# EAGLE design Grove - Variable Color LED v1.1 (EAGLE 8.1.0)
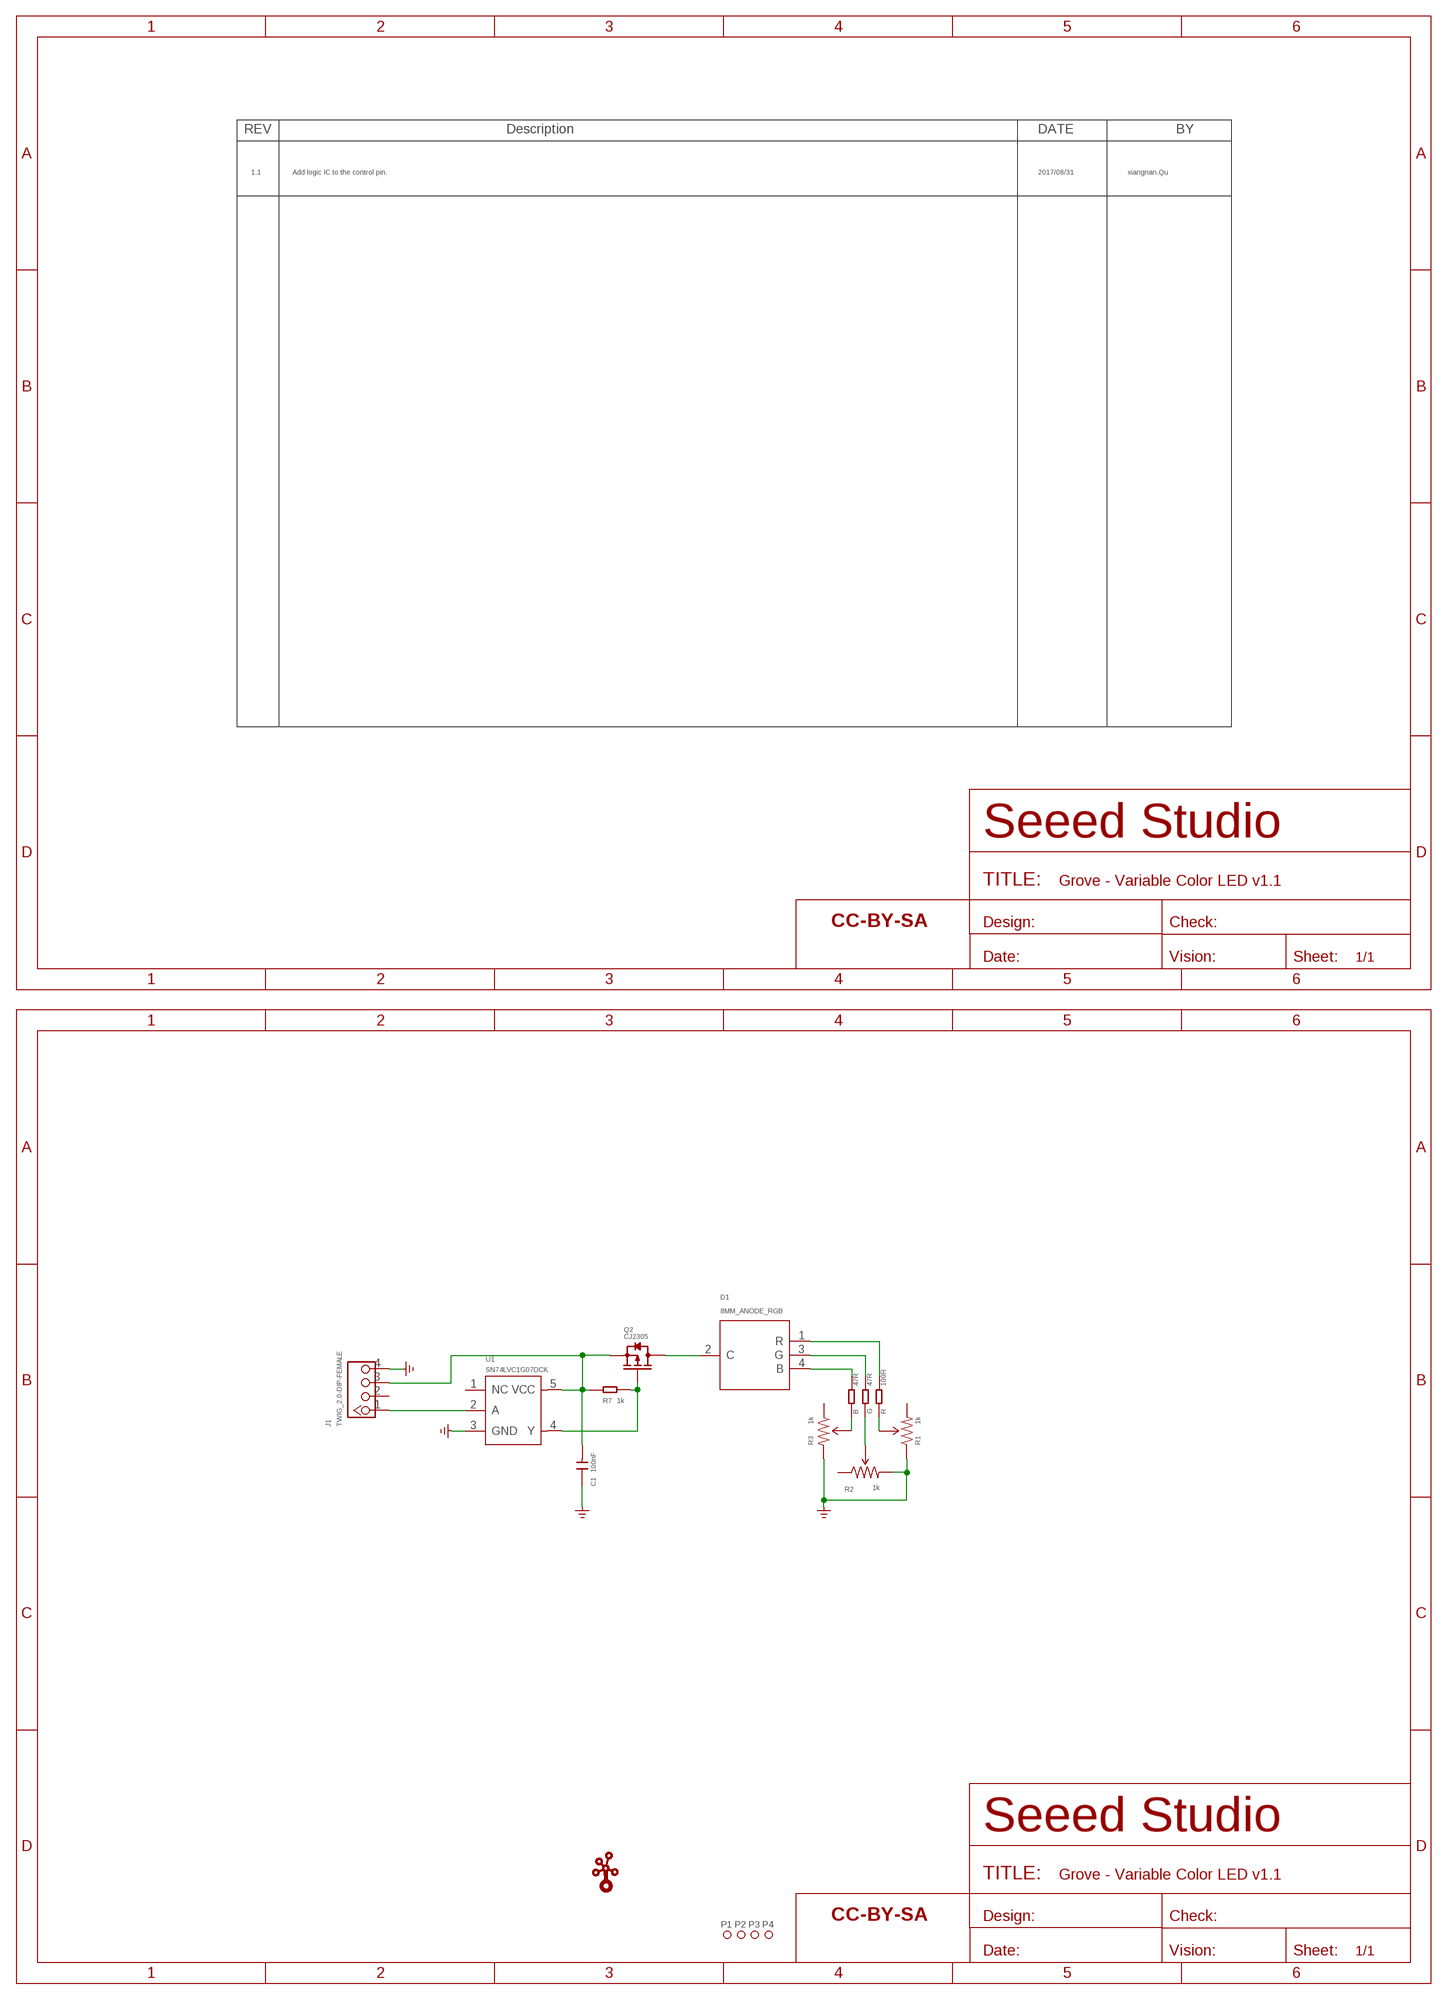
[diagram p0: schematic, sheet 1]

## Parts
B  47R  RES-0402  [R0402]
C1  100nF  CAP-0402  [C0402]
D1  8MM_ANODE_RGB  007-RGB-3P-DIP  [007-RGB-3P-DIP]
FR1  SEEEDSTUDIO-OPEN-SCH-FRAME  [SEEEDSTUDIO-PCB-FRAME]
FR2  SEEEDSTUDIO-OPEN-SCH-FRAME  [SEEEDSTUDIO-PCB-FRAME]
G  47R  RES-0402  [R0402]
J1  TWIG_2.0-DIP-FEMALE  [2.0_1X4]
P1  PAD-MARK'ANNULAR'  [ROUND-MARK-1.0]
P2  PAD-MARK'ANNULAR'  [ROUND-MARK-1.0]
P3  PAD-MARK'ANNULAR'  [ROUND-MARK-1.0]
P4  PAD-MARK'ANNULAR'  [ROUND-MARK-1.0]
Q2  CJ2305  014-P-MOSFETSOT23  [SOT23_]
R  100R  RES-0402  [R0402]
R1  1k  005-TRIMPOTSMD  [TRIMPOT-3MM]
R2  1k  005-TRIMPOTSMD  [TRIMPOT-3MM]
R3  1k  005-TRIMPOTSMD  [TRIMPOT-3MM]
R7  1k  RES-0402  [R0402]
U1  SN74LVC1G07DCK  LOGIC-SN74LVC1G07-DCK  [5P-SMD-2X1.2X1MM]
U$1  TWIGLOGOTWIGLOGO_SMALL  [TWIGLOGO_SMALL]

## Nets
GND: C1.1 J1.4 R1.1(CCW) R2.3(CW) R3.3(CW) U1.3(GND) ; supply symbol labelled GND_POWER
N$1: D1.1(R) R.2
N$2: D1.3(G) G.2
N$3: B.2 D1.4(B)
N$4: G.1 R2.2(WIPER)
N$5: R1.2(WIPER) R.1
N$6: B.1 R3.2(WIPER)
ON/OFF: J1.1 U1.2(A)
RGD_POWER: D1.2(C) Q2.3(D)
SS: Q2.1(G) R7.1 U1.4(Y)
VCC: C1.2 J1.3 Q2.2(S) R7.2 U1.5(VCC)
Unconnected: J1.2 R1.3(CW) R2.1(CCW) R3.1(CCW) U1.1(NC)

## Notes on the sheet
- 1.1 | Add logic IC to the control pin. | 2017/08/31 | xiangnan.Qu

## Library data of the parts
B G R R7 = Discrete-new:RES
C1 = Discrete-new:CAP: Ceramic Capacitors
D1 = Discrete:007-RGB-3P-DIP
FR1 FR2 = moudle-new:SEEEDSTUDIO-OPEN-SCH-FRAME
J1 = Connector:TWIG_2.0-DIP-FEMALE
P1-P4 = Discrete-new:PAD-MARK; PARTNO: DNP
Q2 = Discrete:014-P-MOSFET*: Si2305DS Si2323CDS
R1-R3 = Discrete:005-TRIMPOT
U1 = IC-new:LOGIC-SN74LVC1G07: DRL:310050096 DCK:310050079
U$1 = seeedleo:TWIGLOGO

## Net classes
0 default: width 0.152 mm, drill 0.203 mm, clearance 0.152 mm

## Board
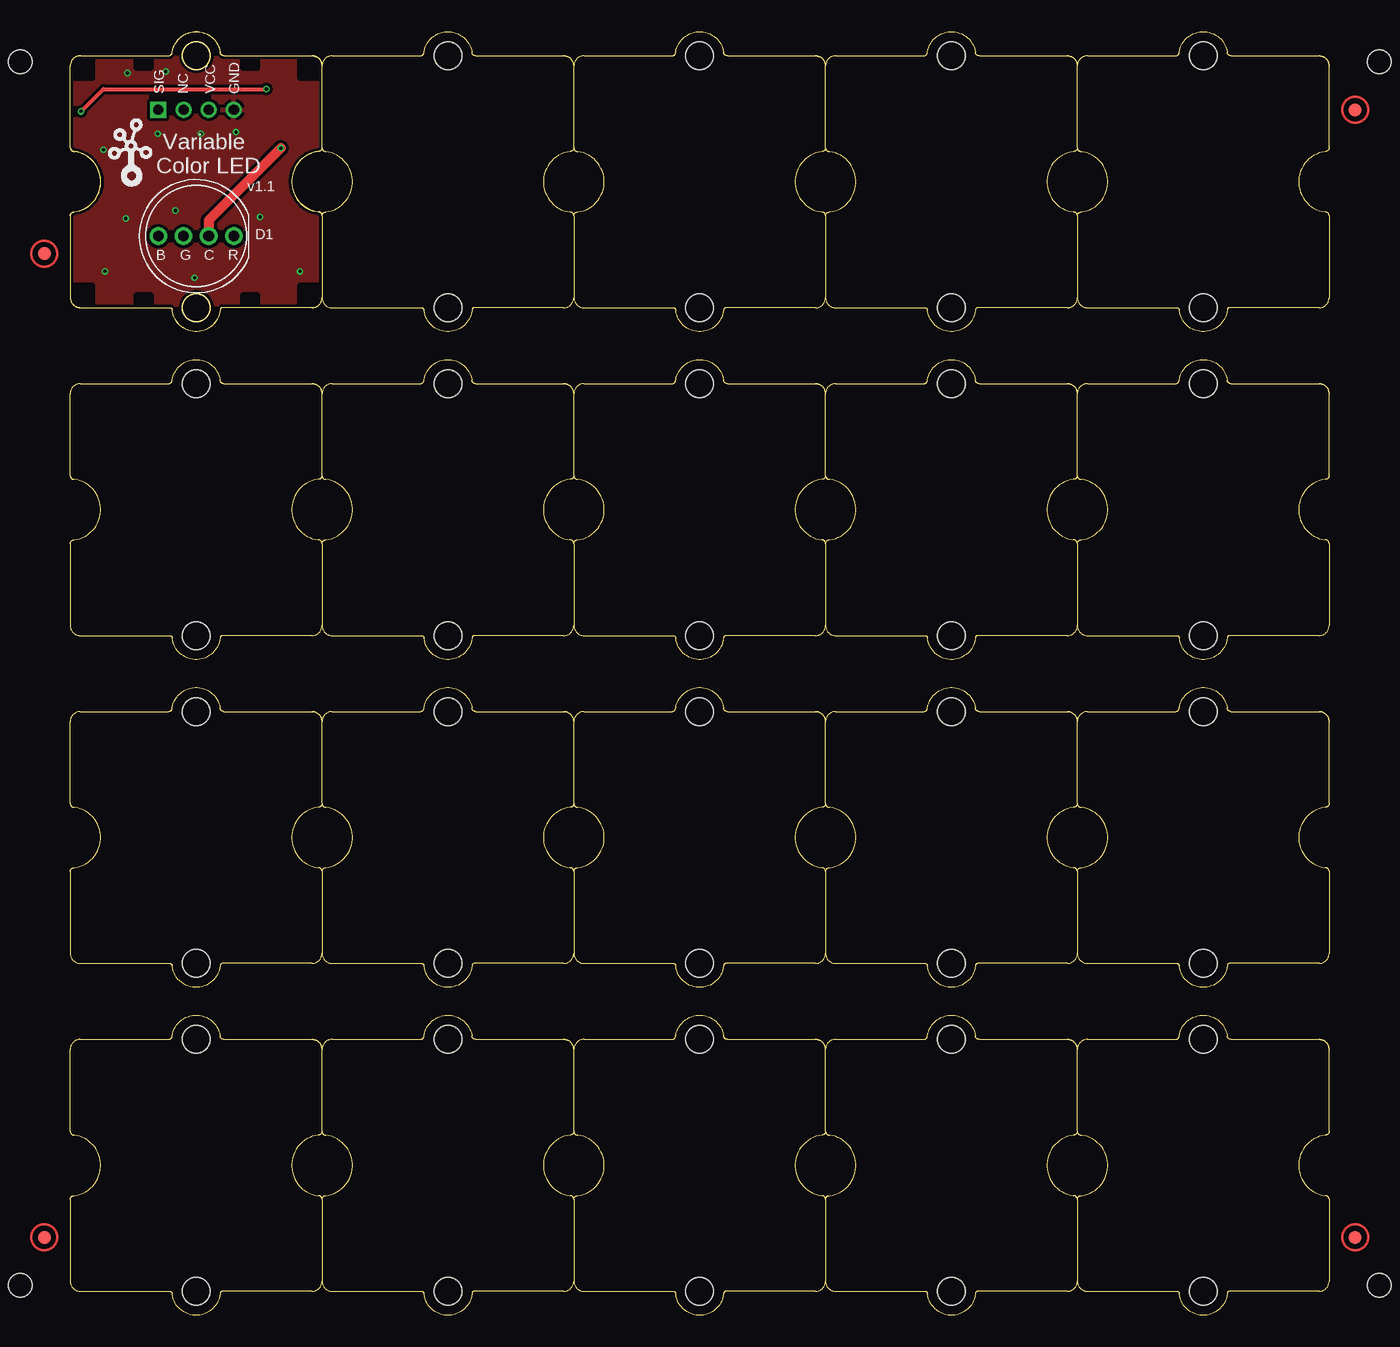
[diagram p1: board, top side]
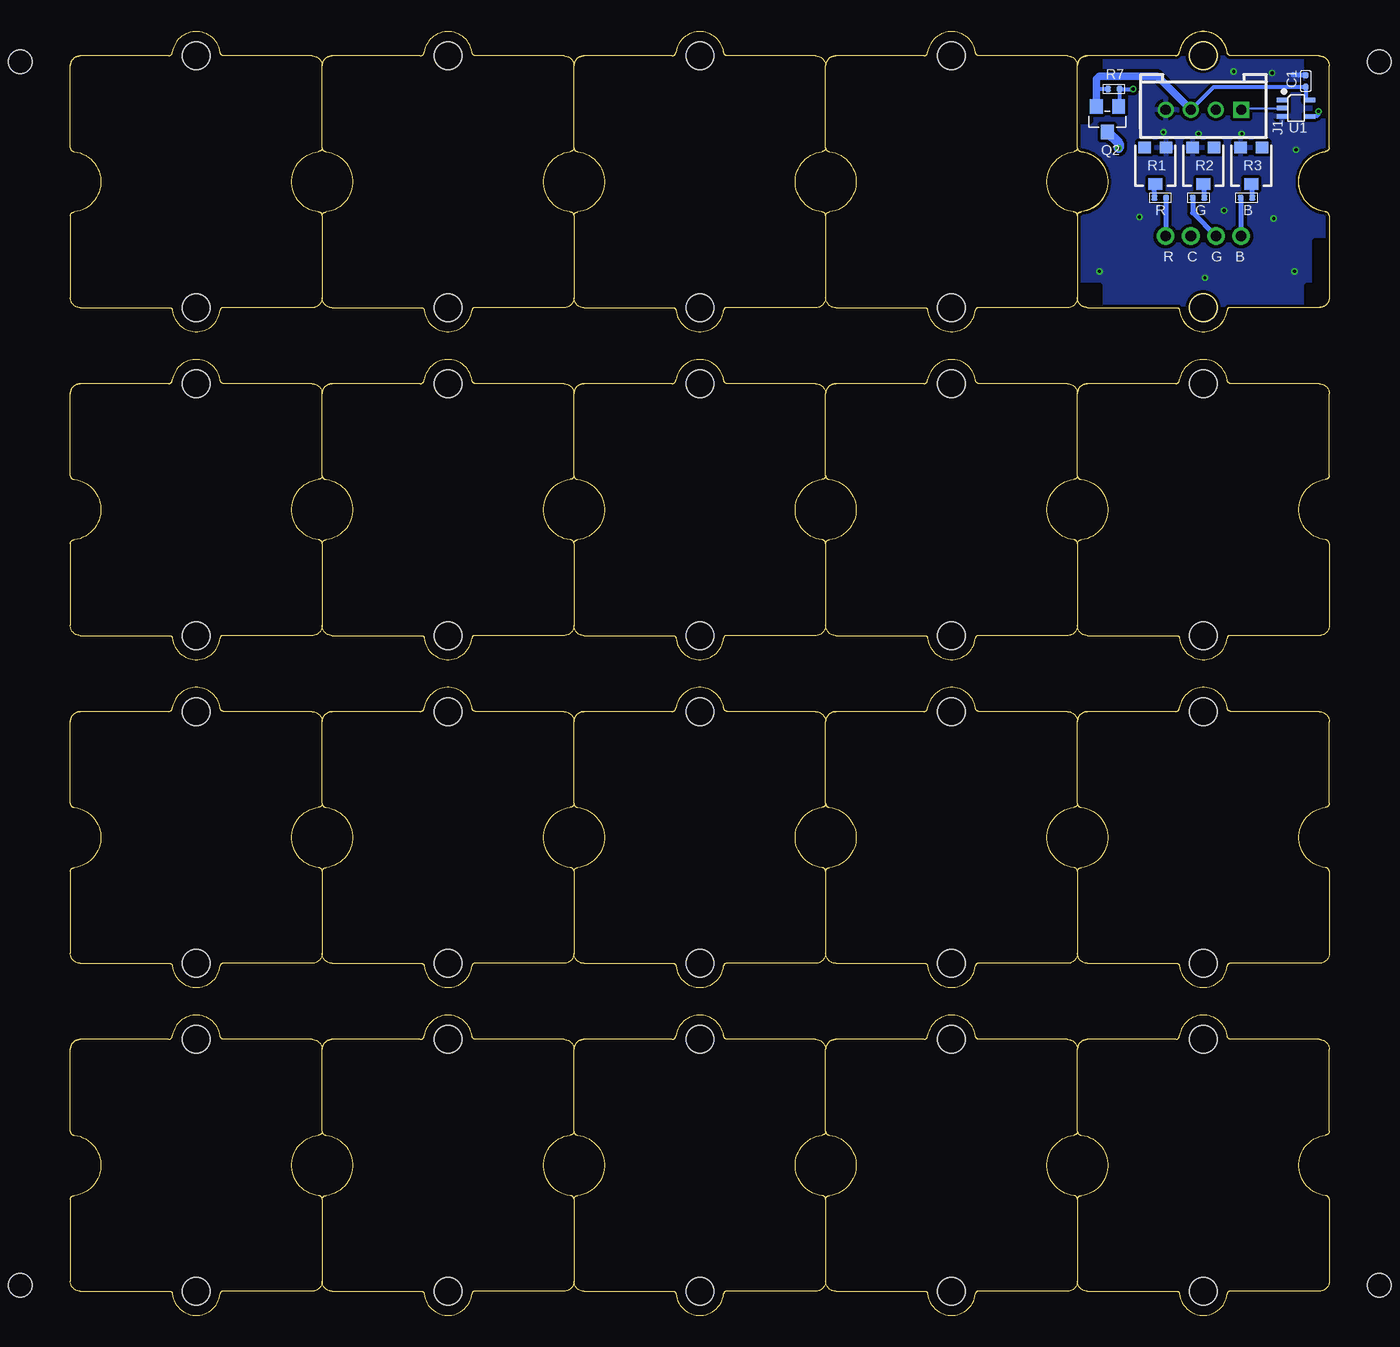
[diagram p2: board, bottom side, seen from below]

Size 100 x 101.95 mm. Coordinates in mm from the lower left corner, seen from the top.
Copper layers (1*2*15*16): Top 0.035mm / dielectric 0.2mm / Route2 0.0175mm / dielectric 0.3mm / Route15 0.0175mm / dielectric 0.2mm / Bottom 0.035mm
Design rules "SeeedStudio_4layer_DRU_no_angle_20140221 *": minimum track width 6mil, minimum drill 8mil, track to track 6mil, track to pad 6mil, pad to pad 6mil, via to via 8mil, smd to smd 0mil, copper to edge 10mil, drill to drill 8mil, minimum pad ring 6mil, minimum via ring 4mil, stop-mask expansion 4mil, vias tented up to drill 25mil, thermal gap 10mil
Holes 1.91 mm at -3.97,2.38 -3.97,99.54 103.98,99.54 103.98,2.38

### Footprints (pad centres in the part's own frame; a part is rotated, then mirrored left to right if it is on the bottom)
R0402 = smd 0.5 x 0.5: 1 0,0.463; 2 0,-0.463
C0402 = smd 0.5 x 0.5: 1 0,0.463; 2 0,-0.463
007-RGB-3P-DIP = drill 0.85 pad 1.4: 1 3,0; 2 1,0; 3 -1,0; 4 -3,0
2.0_1X4 = drill 0.8 pad 1.27 square: 1 -3,0 | drill 0.8 pad 1.27: 2 -1,0; 3 1,0; 4 3,0
ROUND-MARK-1.0 = smd 1.016 x 1.016: P$1 0,0
SOT23_ = smd 1.016 x 1.143: 1 -0.889,-1.016; 2 0.889,-1.016; 3 0,1.016
TRIMPOT-3MM = smd 1 x 0.9: 1 -0.85,-1.45; 3 0.85,-1.45 | smd 1.1 x 0.9: 2 0,1.45
5P-SMD-2X1.2X1MM = smd 0.35 x 0.85: 1 -0.65,-1.1; 2 0,-1.1; 3 0.65,-1.1; 4 0.65,1.1; 5 -0.65,1.1
GROVE-1X1-TEST-PLATFORM-BOTTOM = hole 2.2: 9.987,0.013; -10.013,0.013
GROVE-1*1-TEST-PLATFORM = hole 2.2: 0,-10; 0,10

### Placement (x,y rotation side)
B  6.57,88.74 270 bottom
C1  1.87,98.01 0 bottom
D1  10,85.7 0 top
FR1  not placed on the board
FR2  not placed on the board
G  10.38,88.74 270 bottom
J1  10,95.73 180 bottom
P1  -2.07,6.19 0 top
P2  102.08,6.19 0 top
P3  -2.07,84.3 0 top
P4  102.08,95.73 0 top
Q2  17.62,94.97 180 bottom
R  13.43,88.74 90 bottom
R1  13.81,91.28 180 bottom
R2  10,91.28 180 bottom
R3  6.19,91.28 180 bottom
R7  17.11,97.38 270 bottom
U1  2.63,95.86 270 bottom
U$1  2.63,89.51 0 top
U$5  [GROVE-1X1-TEST-PLATFORM-BOTTOM]  10,90.01 270 top
U$6  [GROVE-1*1-TEST-PLATFORM]  10,90.01 0 top
U$7  [GROVE-1*1-TEST-PLATFORM]  30,90.01 0 top
U$8  [GROVE-1*1-TEST-PLATFORM]  50,90.01 0 top
U$9  [GROVE-1*1-TEST-PLATFORM]  70,90.01 0 top
U$10  [GROVE-1*1-TEST-PLATFORM]  90,90.01 0 top
U$11  [GROVE-1*1-TEST-PLATFORM]  30,63.98 0 top
U$12  [GROVE-1*1-TEST-PLATFORM]  50,63.98 0 top
U$13  [GROVE-1*1-TEST-PLATFORM]  70,63.98 0 top
U$14  [GROVE-1*1-TEST-PLATFORM]  90,63.98 0 top
U$15  [GROVE-1*1-TEST-PLATFORM]  10,63.98 0 top
U$16  [GROVE-1*1-TEST-PLATFORM]  30,37.94 0 top
U$17  [GROVE-1*1-TEST-PLATFORM]  50,37.94 0 top
U$18  [GROVE-1*1-TEST-PLATFORM]  70,37.94 0 top
U$19  [GROVE-1*1-TEST-PLATFORM]  90,37.94 0 top
U$20  [GROVE-1*1-TEST-PLATFORM]  10,37.94 0 top
U$21  [GROVE-1*1-TEST-PLATFORM]  30,11.91 0 top
U$22  [GROVE-1*1-TEST-PLATFORM]  50,11.91 0 top
U$23  [GROVE-1*1-TEST-PLATFORM]  70,11.91 0 top
U$24  [GROVE-1*1-TEST-PLATFORM]  90,11.91 0 top
U$25  [GROVE-1*1-TEST-PLATFORM]  10,11.91 0 top

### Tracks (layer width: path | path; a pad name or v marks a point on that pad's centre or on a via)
GND  (via drill 0.25 pad 0.51)
  Bottom 0.406: C1.1 2.84,98.48 2.89,98.52
  other vias: 13.17,93.95 4.54,98.65 7.59,98.78 2.76,82.9 18.26,82.9 9.87,82.39 15.08,87.22 4.41,87.09 2.63,92.55 8.35,87.73 6.95,93.82 10.38,93.82
  pour Top (isolate 0.254): -0.16,102.08 20.16,102.08 20.16,77.95 -0.16,77.95
  pour Bottom (isolate 0.254): -0.16,102.08 20.16,102.08 20.16,77.95 -0.16,77.95
N$1
  Bottom 0.406: R.2 12.97,85.73 D1.1
N$2
  Bottom 0.406: G.2 10.84,87.54 D1.3
N$3
  Bottom 0.406: D1.4 7,88.71 B.2
N$4
  Bottom 0.406: G.1 9.92,89.75 R2.2
N$5
  Bottom 0.406: R.1 13.94,89.71 R1.2
N$6
  Bottom 0.406: 6.06,89.71 R3.2 6.11,89.75 B.1
ON/OFF
  Bottom 0.152: J1.1 6.87,95.86 U1.2
RGD_POWER  (via drill 0.25 pad 0.51)
  Top 0.813: v16.73,92.68 11,86.95 D1.2
  Bottom 0.813: Q2.3 16.73,93.06 v16.73,92.68
SS  (via drill 0.25 pad 0.51)
  Top 0.305: v0.86,95.6 2.63,97.38 v15.59,97.38
  Bottom 0.305: Q2.1 16.65,96.06 R7.1 v15.59,97.38 | v0.86,95.6 0.86,95.35 0.98,95.22 1.52,95.22 U1.4
VCC
  Bottom 0.152: 18.38,97.38 18.51,97.38
  Bottom 0.305: J1.3 9.18,97.55 C1.2 1.87,96.49 1.55,96.49 U1.5 | R7.2 18.51,97.38
  Bottom 0.61: 18.51,96.95 Q2.2 18.51,97.38 18.51,98.14 18.26,98.4 13.67,98.4 J1.3

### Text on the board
tPlace: SIG | NC | VCC | GND | Variable | Color LED | v1.1
bPlace: B | G | C | R

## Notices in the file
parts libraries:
moudle-new: This work is licensed under the Creative Commons Attribution 4.0 International License.
To view a copy of this license,visit:
http://creativecommons.org/licenses/by-sa/4.0
moudle-new: CC-BY-SA
